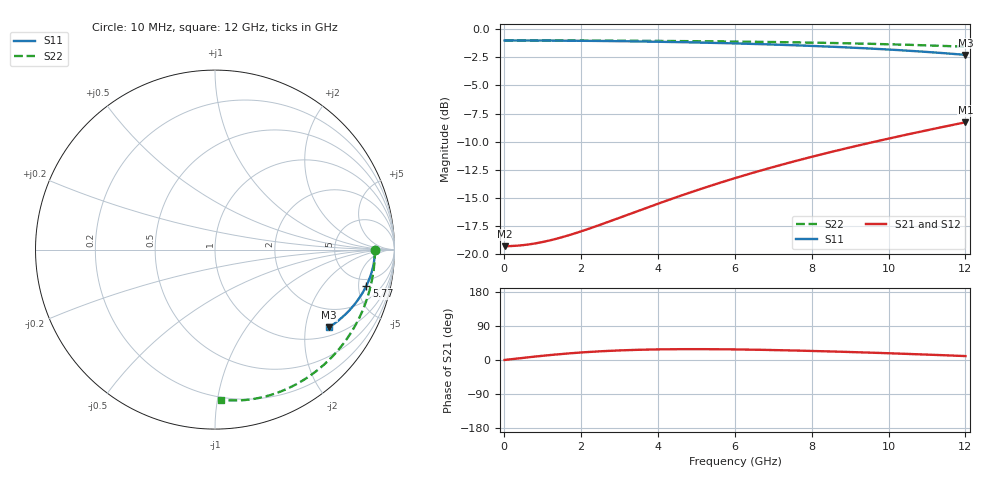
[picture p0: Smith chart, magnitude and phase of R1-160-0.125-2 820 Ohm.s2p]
!version-1
!date-03.2021
# MHz S RI R 50
!Freq ReS11 ImS11 ReS21 ImS21 ReS12 ImS12 ReS22 ImS22
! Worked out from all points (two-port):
!   601 points, 10 MHz to 12 GHz, reference 50 ohm
!   highest |S21| = -8.27 dB at 12 GHz (marker M1); lowest = -19.3 dB at 10 MHz (marker M2)
!   |S21| within 3 dB of the highest: 8.078 GHz to end of sweep
!   lowest |S11| = -2.3 dB at 12 GHz (marker M3), VSWR 7.66, Z = 63.8 - j135 ohm
!   |S11| at or under -10 dB: nowhere
!   |S22| runs from -1.6 to -1.0 dB; largest |S21 - S12| = 0
!   S11 on the Smith chart (normalised r, x): 10 MHz: 17, -0; 5.77 GHz: 3.78, -6.16; 12 GHz: 1.28, -2.70
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10  0.8913 -0.000348  0.1087 0.000221  0.1087 0.000221  0.8913 -0.00138
70  0.8913 -0.00244  0.1087 0.00155  0.1087 0.00155  0.8913 -0.00965
470  0.891 -0.0164  0.1093 0.0104  0.1093 0.0104  0.8889 -0.0647
930  0.8901 -0.0324  0.1109 0.0204  0.1109 0.0204  0.8819 -0.1275
1430  0.8884 -0.0498  0.114 0.0311  0.114 0.0311  0.8693 -0.1947
2010  0.8856 -0.0701  0.1191 0.0431  0.1191 0.0431  0.8482 -0.2705
2490  0.8826 -0.0868  0.1245 0.0526  0.1245 0.0526  0.8259 -0.3309
2970  0.8788 -0.1036  0.131 0.0616  0.131 0.0616  0.7996 -0.3887
3470  0.8742 -0.1212  0.1388 0.0703  0.1388 0.0703  0.7682 -0.4459
4010  0.8684 -0.1402  0.1483 0.0789  0.1483 0.0789  0.7303 -0.5037
4890  0.8569 -0.1713  0.1663 0.0909  0.1663 0.0909  0.661 -0.5884
5770  0.8429 -0.2026  0.1867 0.1002  0.1867 0.1002  0.5848 -0.6604
6010  0.8386 -0.2112  0.1927 0.1022  0.1927 0.1022  0.5632 -0.6779
6510  0.8289 -0.2293  0.2057 0.1057  0.2057 0.1057  0.5172 -0.7111
7010  0.8182 -0.2474  0.2192 0.1082  0.2192 0.1082  0.4704 -0.7402
7510  0.8065 -0.2657  0.2334 0.1096  0.2334 0.1096  0.4233 -0.7653
8010  0.7936 -0.2841  0.2481 0.11  0.2481 0.11  0.3761 -0.7865
8490  0.7801 -0.3019  0.2626 0.1093  0.2626 0.1093  0.331 -0.8032
8990  0.7647 -0.3205  0.2782 0.1075  0.2782 0.1075  0.2847 -0.8172
10010  0.7286 -0.3588  0.3112 0.1001  0.3112 0.1001  0.193 -0.8352
10970  0.688 -0.3949  0.3437 0.0882  0.3437 0.0882  0.1115 -0.8406
12000  0.6357 -0.4328  0.3796 0.0693  0.3796 0.0693  0.0309 -0.8353
